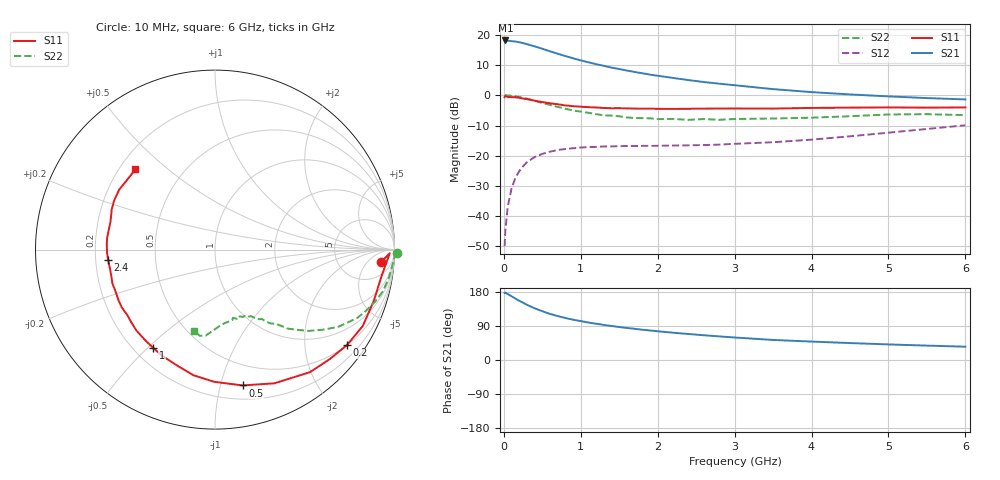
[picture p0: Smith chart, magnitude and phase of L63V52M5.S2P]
!  INFINEON TECHNOLOGIES Small Signal Semiconductors
! BFR380L3 , Si-NPN RF-Transistor in TSLP-3-1
!  Vce=3.5 V,  Ic=2.5 mA
! Common Emitter S-Parameters:  07. March 2005
#  GHz  S  MA  R  50
! f  S11  S21  S12  S22
! GHz  Mag  Ang  Mag  Ang  Mag  Ang  Mag  Ang
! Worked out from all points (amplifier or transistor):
!   36 points, 10 MHz to 6 GHz, reference 50 ohm
!   highest |S21| = 18.1 dB at 20 MHz (marker M1)
!   |S21| within 3 dB of that: start of sweep to 530 MHz
!   unconditionally stable (mu >= 1): 2.76 GHz to 4.616 GHz
!   at 250 MHz: K = 0.09, MSG = 20.4 dB, |S12| = -23.5 dB
!   at 1.4 GHz: K = 0.59, MSG = 13.0 dB, |S12| = -16.9 dB
!   at 6 GHz: K = 0.89, MSG = 4.3 dB, |S12| = -9.9 dB
!   S11 on the Smith chart (normalised r, x): 10 MHz: 13, -13; 200 MHz: 0.50, -3.01; 500 MHz: 0.31, -1.17; 1 GHz: 0.28, -0.52; 2.4 GHz: 0.25, -0.04; 6 GHz: 0.26, +0.39
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0.01  0.9277 -4.3  8.007 177.1  0.0032 85.1  1.014 -1.0
0.02  0.9739 -1.2  8.062 177.9  0.0059 87.7  1.003 -2.0
0.05  0.9392 -9.2  7.969 174.0  0.0142 87.9  0.9931 -4.7
0.1  0.9298 -17.8  7.844 168.2  0.0288 79.8  0.981 -9.4
0.15  0.927 -27.3  7.748 162.2  0.0431 75.4  0.9634 -14.0
0.2  0.9076 -35.9  7.525 156.3  0.0556 71.5  0.9388 -17.9
0.3  0.864 -52.2  7.001 145.7  0.0781 62.9  0.8789 -25.7
0.4  0.8151 -66.1  6.449 136.5  0.0952 55.9  0.8101 -32.1
0.5  0.7722 -78.5  5.875 128.8  0.1074 50.5  0.7474 -36.7
0.6  0.7367 -90.3  5.335 121.6  0.1167 45.9  0.6919 -40.9
0.7  0.7103 -99.7  4.861 116.0  0.1246 42.9  0.6427 -44.1
0.9  0.6607 -116.4  4.088 106.3  0.133 37.4  0.5595 -49.2
1  0.6474 -122.1  3.772 102.7  0.1368 36.1  0.5374 -50.5
1.1  0.6357 -128.6  3.507 98.8  0.1388 34.6  0.5137 -53.1
1.3  0.6172 -139.3  3.071 92.6  0.1426 33.3  0.4665 -55.9
1.6  0.6069 -152.6  2.563 84.5  0.145 32.6  0.4298 -60.7
2.2  0.5947 -169.7  1.935 72.0  0.1478 35.6  0.4065 -67.3
2.4  0.5983 -174.5  1.783 68.6  0.1487 37.4  0.3927 -70.9
3.5  0.6029 164.8  1.264 52.9  0.1674 49.4  0.4129 -82.4
4.5  0.6252 153.9  1.033 44.7  0.2097 60.2  0.4506 -91.2
5.5  0.6251 141.6  0.899 38.0  0.2773 64.6  0.4875 -100.0
6  0.6297 134.8  0.854 35.1  0.3191 64.4  0.4695 -104.5
